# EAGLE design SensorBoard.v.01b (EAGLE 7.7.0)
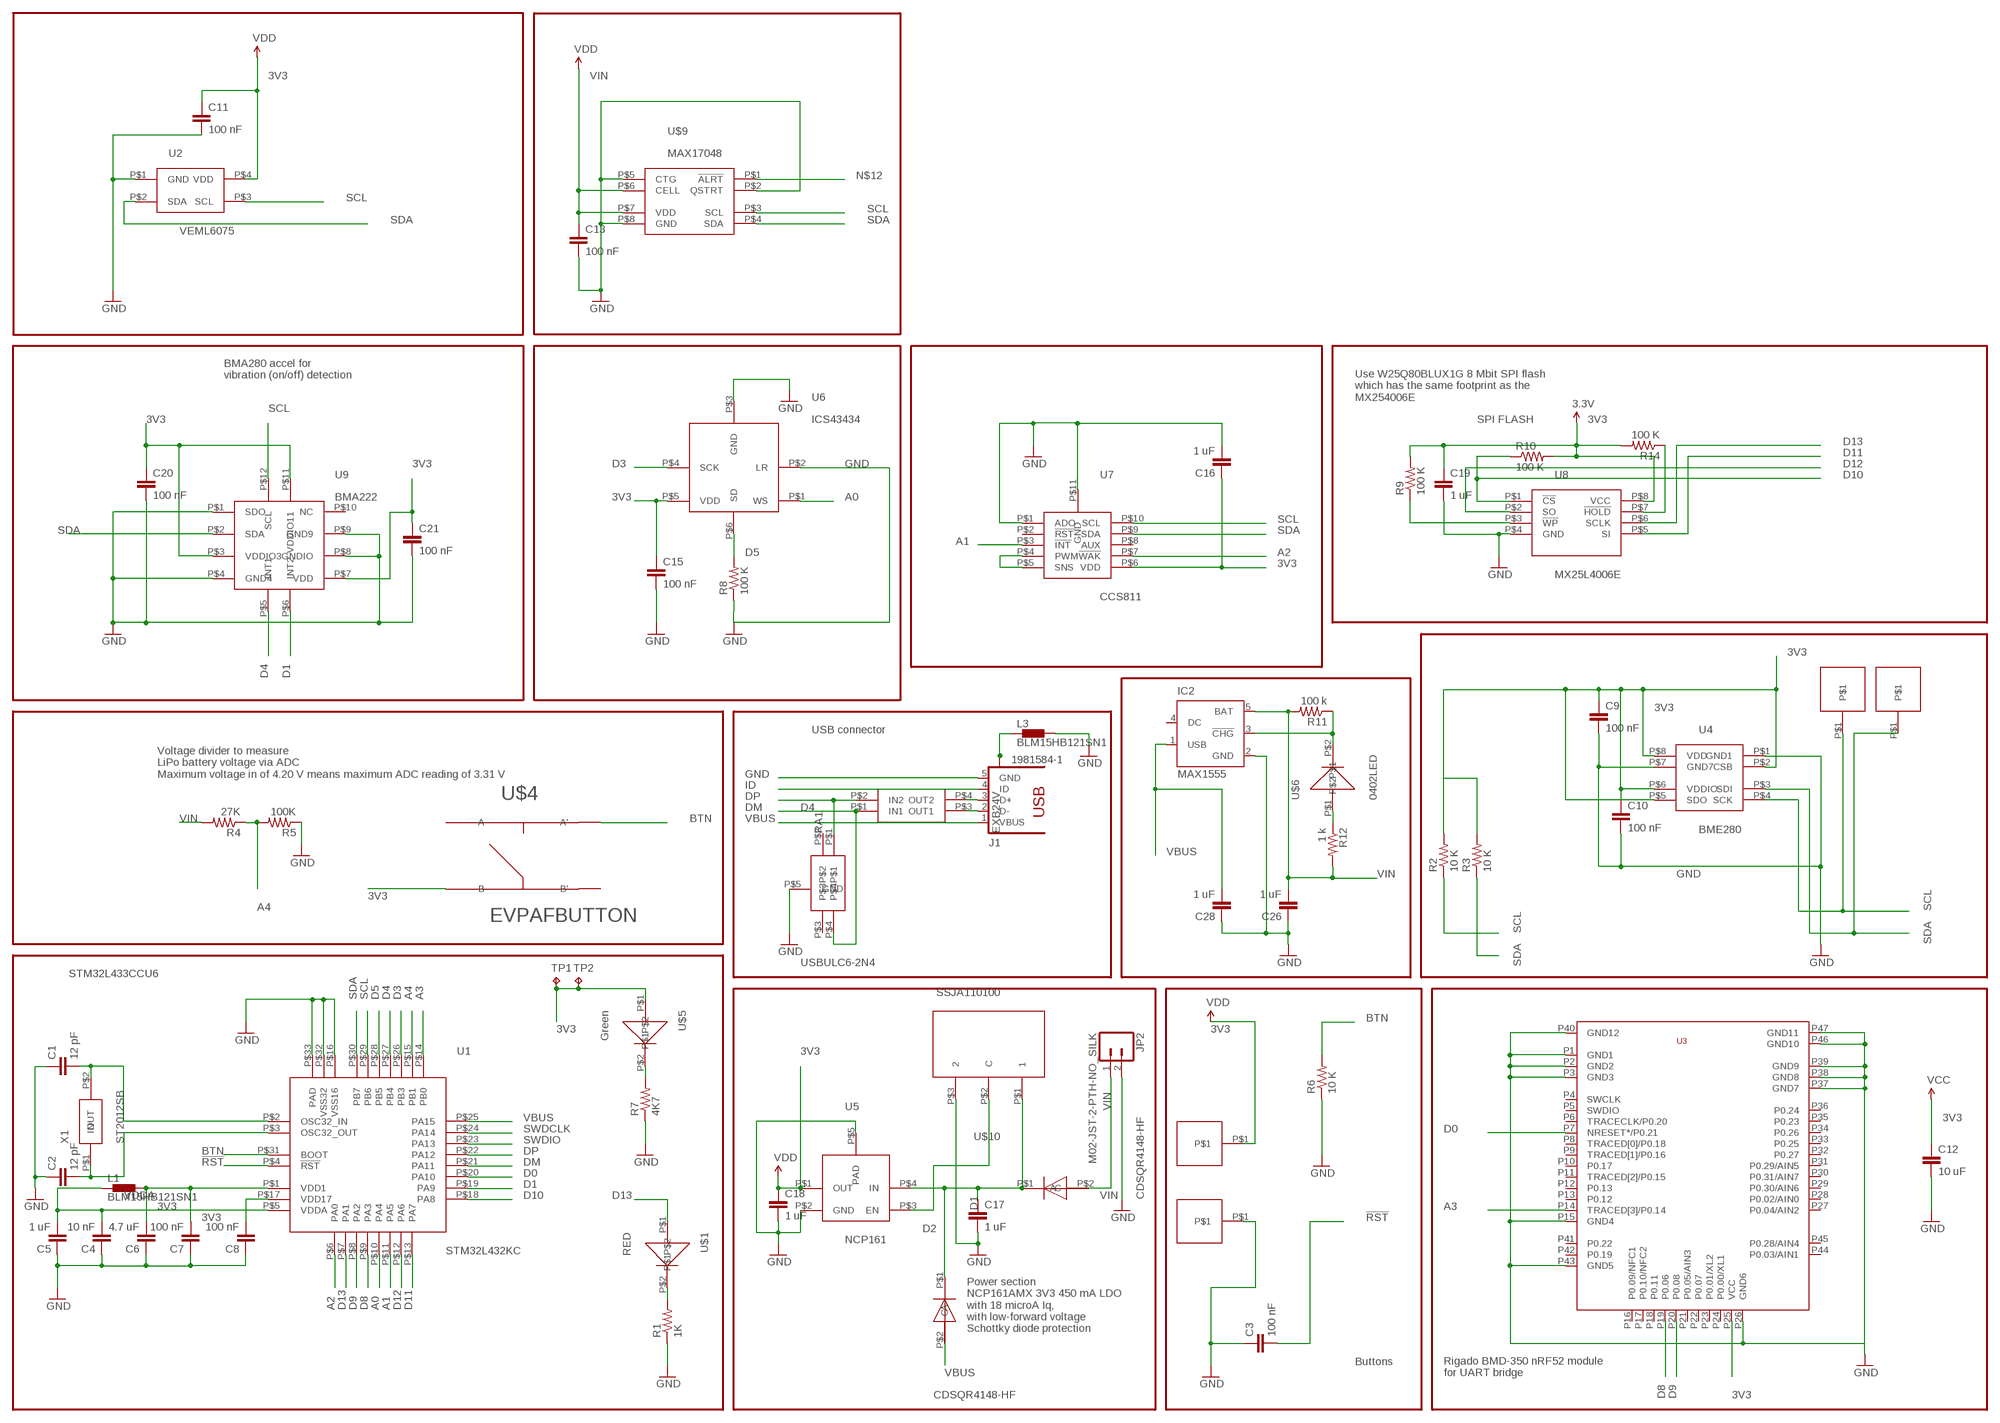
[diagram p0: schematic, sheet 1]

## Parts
C1  12 pF  0402CAP.KW  [0402-CAP]
C2  12 pF  0402CAP.KW  [0402-CAP]
C3  100 nF  0402CAP.KW  [0402-CAP]
C4  10 nF  0402CAP.KW  [0402-CAP]
C5  1 uF  0402CAP.KW  [0402-CAP]
C6  4.7 uF  0402CAP.KW  [0402-CAP]
C7  100 nF  0402CAP.KW  [0402-CAP]
C8  100 nF  0402CAP.KW  [0402-CAP]
C9  100 nF  CAP0402-CAP  [0402-CAP]
C10  100 nF  CAP0402-CAP  [0402-CAP]
C11  100 nF  0402CAP.KW  [0402-CAP]
C12  10 uF  CAP0402-CAP  [0402-CAP]
C13  100 nF  0402CAP.KW  [0402-CAP]
C15  100 nF  0402CAP.KW  [0402-CAP]
C16  1 uF  0402CAP.KW  [0402-CAP]
C17  1 uF  0402CAP.KW  [0402-CAP]
C18  1 uF  0402CAP.KW  [0402-CAP]
C19  1 uF  0402CAP.KW  [0402-CAP]
C20  100 nF  CAP0402-CAP  [0402-CAP]
C21  100 nF  CAP0402-CAP  [0402-CAP]
C26  1 uF  0402CAP.KW  [0402-CAP]
C28  1 uF  0402CAP.KW  [0402-CAP]
D1  CDSQR4148-HF  [CDSQR4148-HF]
D2  CDSQR4148-HF  [CDSQR4148-HF]
D4  USBULC6-2N4  [USBULC6-2N4]
IC2  MAX1555  [SOT23-5L]
J1  1981584-1  [1981584-1]
JP2  M02-JST-2-PTH-NO_SILK  [JST-2-PTH-NS]
L1  BLM15HB121SN1  [0402]
L3  BLM15HB121SN1  [0402]
R1  1K  0402RES.KW  [0402-RES]
R2  10 K  0402RES.KW  [0402-RES]
R3  10 K  0402RES.KW  [0402-RES]
R4  27K  0402RES.KW  [0402-RES]
R5  100K  0402RES.KW  [0402-RES]
R6  10 K  0402RES.KW  [0402-RES]
R7  4K7  0402RES.KW  [0402-RES]
R8  100 K  0402RES.KW  [0402-RES]
R9  100 K  0402RES.KW  [0402-RES]
R10  100 K  0402RES.KW  [0402-RES]
R11  100 k  0402RES.KW  [0402-RES]
R12  1 k  0402RES.KW  [0402-RES]
R14  100 K  0402RES.KW  [0402-RES]
RA1  EXB24V  [EXB24V]
TP1  TPTP06SQ  [TP06SQ]
TP2  TPTP06SQ  [TP06SQ]
U1  STM32L432KC  [STM32L432KC]
U2  VEML6075  [A3OP]
U3  BMD-350  [BMD-350]
U4  BME280  [BME280]
U5  NCP161  [NCP161]
U6  ICS43434  [ICS43434]
U7  CCS811  [CCS811]
U8  MX25L4006E  [USON-8]
U9  BMA222  [BMA222]
U$1  RED  0402LED  [0402LED]
U$2  HN01  [HN01]
U$3  HN01  [HN01]
U$4  EVPAFBUTTON  [EVPAF-BUTTON-SPDT]
U$5  Green  0402LED  [0402LED]
U$6  0402LED  [0402LED]
U$7  HN01  [HN01]
U$8  HN01  [HN01]
U$9  MAX17048  [MAX17048]
U$10  SSJA110100  [SSAJ110100]
X1  ST2012SB  [ST2012SB]

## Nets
3V3: C6.2 C7.2 C8.2 C9.1 C10.1 C11.1 C12.1 C15.1 C16.1 C18.1 C19.1 C20.1 C21.1 L1.2 R2.2 R3.2 R9.2 R10.2 R14.2 TP1.TP TP2.TP U1.P$1(VDD1) U1.P$17(VDD17) U2.P$4(VDD) U3.P25(VCC) U4.P$2(CSB) U4.P$5(SDO) U4.P$6(VDDIO) U4.P$8(VDD) U5.P$1(OUT) U6.P$5(VDD) U7.P$6(VDD) U8.P$8(VCC) U9.P$3(VDDIO3) U9.P$7(VDD) U9.P$11(VDDIO11) U$2.P$1 U$4.P$3(B) U$5.P$1 ; supply symbol labelled VDD, VCC, 3.3V
!RST: C3.2 U1.P$4(!RST)
A0: U1.P$10(PA4) U6.P$1(WS)
A1: U1.P$11(PA5) U7.P$3(!INT)
A2: U1.P$6(PA0) U7.P$7(!WAK)
A3: U1.P$14(PB0) U3.P14(TRACED[3]/P0.14)
A4: R4.1 R5.2 U1.P$15(PB1)
BTN: R6.2 U1.P$31(BOOT) U$4.P$2(A')
D0: U1.P$20(PA10) U3.P7(NRESET*/P0.21)
D1: U1.P$19(PA9) U9.P$6(INT2)
D3: U1.P$26(PB3) U6.P$4(SCK)
D4: U1.P$27(PB4) U9.P$5(INT1)
D5: R8.2 U1.P$28(PB5) U6.P$6(SD)
D8: U1.P$9(PA3) U3.P19(P0.06)
D9: U1.P$8(PA2) U3.P20(P0.08)
D10: R10.1 U1.P$18(PA8) U8.P$1(!CS)
D11: U1.P$13(PA7) U8.P$5(SI)
D12: U1.P$12(PA6) U8.P$2(SO)
D13: U1.P$7(PA1) U8.P$6(SCLK) U$1.P$1
DM: D4.P$4 RA1.P$1(IN1) U1.P$21(PA11)
DP: D4.P$1 RA1.P$2(IN2) U1.P$22(PA12)
GND: C1.1 C2.1 C3.1 C4.1 C5.1 C6.1 C7.1 C8.1 C9.2 C10.2 C11.2 C12.2 C13.2 C15.2 C16.2 C17.2 C18.2 C19.2 C20.2 C21.2 C26.1 C28.1 D4.P$5(GND) IC2.2(GND) J1.5(GND) JP2.2 L3.2 R1.1 R5.1 R6.1 R7.1 R8.1 U1.P$16(VSS16) U1.P$32(VSS32) U1.P$33(PAD) U2.P$1(GND) U3.P1(GND1) U3.P2(GND2) U3.P3(GND3) U3.P15(GND4) U3.P26(GND6) U3.P37(GND7) U3.P38(GND8) U3.P39(GND9) U3.P40(GND12) U3.P43(GND5) U3.P46(GND10) U3.P47(GND11) U4.P$1(GND1) U4.P$7(GND7) U5.P$2(GND) U5.P$5(PAD) U6.P$2(LR) U6.P$3(GND) U7.P$1(ADO) U7.P$11(GND) U8.P$4(GND) U9.P$1(SDO) U9.P$4(GND4) U9.P$8(GNDIO) U9.P$9(GND9) U$3.P$1 U$9.P$2(QSTRT) U$9.P$5(CTG) U$9.P$8(GND) U$10.P$3
ID: J1.4(ID)
N$1: R1.2 U$1.P$2
N$2: U5.P$3(EN) U$10.P$2(C)
N$3: C1.2 U1.P$2(OSC32_IN) X1.P$2(OUT)
N$4: C2.2 U1.P$3(OSC32_OUT) X1.P$1(IN)
N$7: R7.2 U$5.P$2
N$10: U7.P$4(PWM) U7.P$5(SNS)
N$12: U$9.P$1(!ALRT)
N$20: R9.1 U8.P$3(!WP)
N$21: R14.1 U8.P$7(!HOLD)
N$31: J1.3(D+) RA1.P$4(OUT2)
N$33: J1.2(D-) RA1.P$3(OUT1)
N$43: R12.1 U$6.P$1
N$48: IC2.3(!CHG) R11.1 U$6.P$2
N$60: C17.1 D1.P$1(C) D2.P$1(C) U5.P$4(IN) U$10.P$1
SCL: R2.1 U1.P$29(PB6) U2.P$3(SCL) U4.P$4(SCK) U7.P$10(SCL) U9.P$12(SCL) U$7.P$1 U$9.P$3(SCL)
SDA: R3.1 U1.P$30(PB7) U2.P$2(SDA) U4.P$3(SDI) U7.P$9(SDA) U9.P$2(SDA) U$8.P$1 U$9.P$4(SDA)
SWDCLK: U1.P$24(PA14)
SWDIO: U1.P$23(PA13)
USB_SHIELD: J1.S1 J1.S2 J1.S3 J1.S4 L3.1
VBUS: C28.2 D2.P$2(A) IC2.1(USB) J1.1(VBUS) U1.P$25(PA15)
VDDA: C4.2 C5.2 L1.1 U1.P$5(VDDA)
VIN: C13.1 C26.2 D1.P$2(A) IC2.5(BAT) JP2.1 R4.2 R11.2 R12.2 U$9.P$6(CELL) U$9.P$7(VDD) ; supply symbol labelled VDD
Unconnected: D4.P$2 D4.P$3 IC2.4(DC) U3.P4(SWCLK) U3.P5(SWDIO) U3.P6(TRACECLK/P0.20) U3.P8(TRACED[0]/P0.18) U3.P9(TRACED[1]/P0.16) U3.P10(P0.17) U3.P11(TRACED[2]/P0.15) U3.P12(P0.13) U3.P13(P0.12) U3.P16(P0.09/NFC1) U3.P17(P0.10/NFC2) U3.P18(P0.11) U3.P21(P0.05/AIN3) U3.P22(P0.07) U3.P23(P0.01/XL2) U3.P24(P0.00/XL1) U3.P27(P0.04/AIN2) U3.P28(P0.02/AIN0) U3.P29(P0.30/AIN6) U3.P30(P0.31/AIN7) U3.P31(P0.29/AIN5) U3.P32(P0.27) U3.P33(P0.25) U3.P34(P0.26) U3.P35(P0.23) U3.P36(P0.24) U3.P41(P0.22) U3.P42(P0.19) U3.P44(P0.03/AIN1) U3.P45(P0.28/AIN4) U7.P$2(!RST) U7.P$8(AUX) U9.P$10(NC) U$4.P$1(A) U$4.P$4(B')

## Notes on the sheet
- BMA280 accel for
  vibration (on/off) detection
- Use W25Q80BLUX1G 8 Mbit SPI flash 
  which has the same footprint as the 
  MX254006E
- SPI FLASH
- USB connector
- Voltage divider to measure 
  LiPo battery voltage via ADC
  Maximum voltage in of 4.20 V means maximum ADC reading of 3.31 V
- STM32L433CCU6
- Power section
  NCP161AMX 3V3 450 mA LDO
  with 18 microA Iq, 
  with low-forward voltage 
  Schottky diode protection
- Buttons
- Rigado BMD-350 nRF52 module
  for UART bridge

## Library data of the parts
C1-C8 C11 C13 C15-C19 C26 C28 = SparkFun-Capacitors:0402CAP.KW
C9 C10 C12 C20 C21 = SparkFun-Capacitors:CAP: Capacitor
D1 D2 = Kris:CDSQR4148-HF: ComChip's CDSQR4148-HF high speed 150 mA Io diode
D4 = Kris:USBULC6-2N4: ST TVS diode ESD Protection USBULC6-2N4
IC2 = maxim:MAX1555: Dual-Input USB/AC Adapter 1-Cell Li+ Battery Chargers Source: http://www.maxim-ic.com .. MAX1551-MAX1555.pdf; MF: MAXIM; MPN: MAX1555EZK+T; OC_FARNELL: 1628222; OC_NEWARK: 59J2761
J1 = con-usb:1981584-1: Receptacle, micro-USB, type A/B Tyco Electronics; MF: Hirose; MPN: ZX62-AB-5PA(11)
JP2 = SparkFun-Connectors:M02: Standard 2-pin 0.1" header. Use with
L1 L3 = inductors:BLM15H: EMIFIL (R) Chip Ferrite Bead for GHz Noise
R1-R12 R14 = SparkFun-Resistors:0402RES.KW
RA1 = Kris:EXB24V: Panasonic EXB24 22 Ohm series resistor pair
TP1 TP2 = testpad:TP: Test pad
U1 = STM32L432KC:STM32L432KC: STM32L432KC UFQFPN32 - 32-pin, 5x5 mm, 0.5 mm pitch ultra thin fine pitch quad flat package http://www.st.com/content/ccc/resource/technical/document/datasheet/24/01/9f/59/f0/83/47/fc/DM00257205.pdf/files/DM00257205.pdf/jcr:content/translations/en.DM00257205.pdf
U2 = Kris:VEML6075: A3OP package for VEML6040 and VEML6075 Vishay light sensors
U3 = BMD-350-Eagle:BMD-350
U4 = Kris:BME280: BME280 Bosch pressure, humidity, temperature sensor
U5 = Kris:NCP161: NCP161 3V3 LDO voltage regulator
U6 = Invensense:ICS43434: ICS43434 I2S Digital Microphone
U7 = Kris:CCS811: CCS811 Air Quality Sensor http://ams.com/eng/Products/Environmental-Sensors/Gas-Sensors/CCS811
U8 = Kris:MX25L4006E: uson-8 package for Macronix MX25L4006E 4 Mbit SPI Fash
U9 = Kris:BMA222: Bosch BMA222 3-axis accelerometer
U$1 U$5 U$6 = Kris:0402LED: 0402led
U$2 U$3 U$7 U$8 = PWSONN6:HN01
U$4 = SparkFun-Electromechanical:EVPAFBUTTON: EVPAF Momentary switch by panasonic
U$9 = Kris:MAX17048: MAX17048 LiPo Battery Fuel Gauge
U$10 = Kris:SSJA110100: ALPS SSJA110100 SPDT slide switch with lugs
X1 = Kris:ST2012SB: Kyocera 2.0 x 1.2 mm 32.768 20kHz ppm 4 pf crystal

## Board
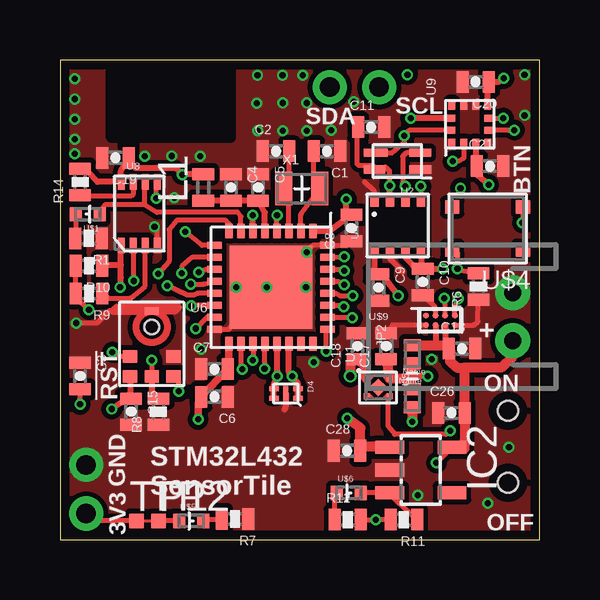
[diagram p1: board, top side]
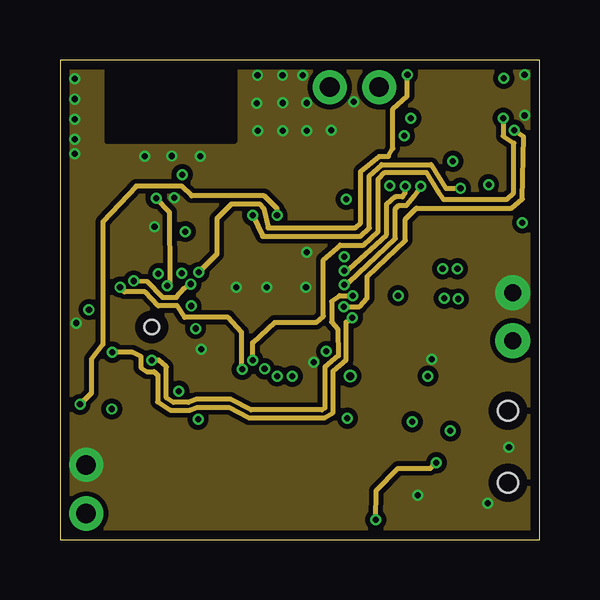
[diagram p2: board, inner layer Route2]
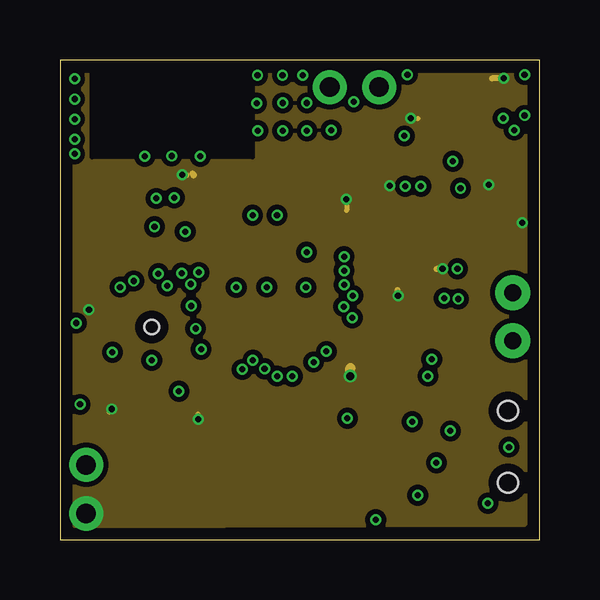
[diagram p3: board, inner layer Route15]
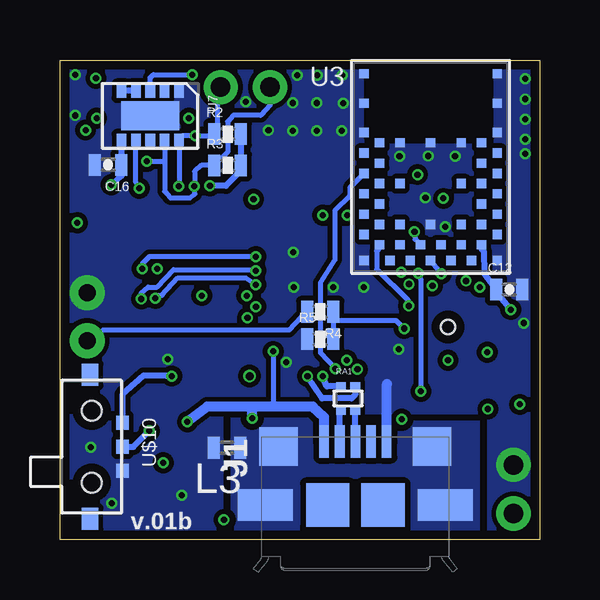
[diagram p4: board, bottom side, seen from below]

Size 19.99 x 19.99 mm. Coordinates in mm from the lower left corner, seen from the top.
Outline: 0,0 19.99,0 19.99,19.99 0,19.99 0,0
Copper layers (1*2*15*16): Top 0.035559375mm / dielectric 0.17018125mm / Route2 0.01778125mm / dielectric 47mil / Route15 0.01778125mm / dielectric 0.17018125mm / Bottom 0.035559375mm
Design rules "OSHPark-4layer *": minimum track width 5mil, minimum drill 10mil, track to track 5mil, track to pad 5mil, pad to pad 5mil, via to via 5mil, smd to smd 5mil, copper to edge 15mil, drill to drill 6mil, minimum pad ring 4mil, minimum via ring 4mil, stop-mask expansion 4mil, vias tented up to drill 20mil, thermal gap 10mil

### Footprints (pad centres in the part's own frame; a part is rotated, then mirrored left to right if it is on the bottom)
0402-CAP = smd 0.5 x 0.9: 1 -0.55,0; 2 0.55,0
CDSQR4148-HF = smd 0.7 x 0.5: P$1 0,0.375; P$2 0,-0.375
USBULC6-2N4 = smd 0.2 x 0.4: P$1 0.2,0.5; P$2 -0.2,0.5; P$3 -0.2,-0.5; P$4 0.2,-0.5 | smd 0.6 x 0.2: P$5 0,0
SOT23-5L = smd 0.55 x 1.2: 1 -0.95,-1.3; 2 0,-1.3; 3 0.95,-1.3; 4 0.95,1.3; 5 -0.95,1.3
1981584-1 = smd 0.4 x 1.35: 1 -1.3,4.1; 2 -0.65,4.1; 3 0,4.1; 4 0.65,4.1; 5 1.3,4.1 | smd 1.8 x 1.8: M1 -1.15,1.45; M2 1.15,1.45 | smd 2.3 x 1.3: S1 -3.75,1.45; S2 3.75,1.45 | smd 1.6 x 1.6: S3 -3.2,3.885; S4 3.2,3.885
JST-2-PTH-NS = drill 0.7 pad 1.448: 1 -1,0; 2 1,0
0402 = smd 0.5 x 0.9: 1 -0.55,0; 2 0.55,0
0402-RES = smd 0.5 x 0.9: 1 -0.55,0; 2 0.55,0
EXB24V = smd 0.4 x 0.36: P$1 -0.3,0.5; P$2 0.3,0.5; P$3 -0.3,-0.5; P$4 0.3,-0.5
TP06SQ = smd 0.6 x 0.6: TP 0,0
STM32L432KC = smd 0.6 x 0.3: P$1 -2.35,1.75; P$2 -2.35,1.25; P$3 -2.35,0.75; P$4 -2.35,0.25; P$5 -2.35,-0.25; P$6 -2.35,-0.75; P$7 -2.35,-1.25; P$8 -2.35,-1.75; P$17 2.35,-1.75; P$18 2.35,-1.25; P$19 2.35,-0.75; P$20 2.35,-0.25; P$21 2.35,0.25; P$22 2.35,0.75; P$23 2.35,1.25; P$24 2.35,1.75 | smd 0.3 x 0.6: P$9 -1.75,-2.35; P$10 -1.25,-2.35; P$11 -0.75,-2.35; P$12 -0.25,-2.35; P$13 0.25,-2.35; P$14 0.75,-2.35; P$15 1.25,-2.35; P$16 1.75,-2.35; P$25 1.75,2.35; P$26 1.25,2.35; P$27 0.75,2.35; P$28 0.25,2.35; P$29 -0.25,2.35; P$30 -0.75,2.35; P$31 -1.25,2.35; P$32 -1.75,2.35 | smd 3.45 x 3.45: P$33 0,0
A3OP = smd 0.9 x 0.35: P$1 -0.95,0.35; P$2 -0.95,-0.35; P$4 0.95,0.35 | smd 1 x 0.35: P$3 0.9,-0.35
BMD-350 = smd 0.39 x 0.39: P1 0.425,8.2; P2 0.425,6.975; P3 0.425,5.75; P4 1.075,5.325; P5 0.425,4.9; P6 1.075,4.475; P7 0.425,4.05; P8 1.075,3.625; P9 0.425,3.2; P10 1.075,2.775; P11 0.425,2.35; P12 1.075,1.925; P13 0.425,1.5; P14 1.075,1.075; P15 0.425,0.425; P16 1.5,0.425; P17 1.925,1.075; P18 2.35,0.425; P19 2.775,1.075; P20 3.2,0.425; P21 3.625,1.075; P22 4.05,0.425; P23 4.475,1.075; P24 4.9,0.425; P25 5.325,1.075; P26 5.975,0.425; P27 5.975,1.5; P28 5.325,1.925; P29 5.975,2.35; P30 5.325,2.775; P31 5.975,3.2; P32 5.325,3.625; P33 5.975,4.05; P34 5.325,4.475; P35 5.975,4.9; P36 5.325,5.325; P37 5.975,5.75; P38 5.975,6.975; P39 5.975,8.2; P40 1.925,5.325; P41 1.925,3.625; P42 1.925,1.925; P43 3.2,1.925; P44 4.475,1.925; P45 4.475,3.625; P46 4.475,5.325; P47 3.2,5.325
BME280 = smd 0.5 x 0.35: P$1 1.025,0.975; P$2 1.025,0.325; P$3 1.025,-0.325; P$4 1.025,-0.975; P$5 -1.025,-0.975; P$6 -1.025,-0.325; P$7 -1.025,0.325; P$8 -1.025,0.975
NCP161 = smd 0.24 x 0.24: P$1 -0.37,-0.48; P$2 0.37,-0.48; P$3 0.37,0.48; P$4 -0.37,0.48 | smd 0.52 x 0.52 rotated 45: P$5 0,0
ICS43434 = smd 0.6 x 0.522: P$1 0.9,-1.364; P$2 0.9,-0.532; P$4 -0.9,-0.532; P$5 -0.9,-1.364; P$6 0,-1.364 | smd 0.6 x 0.3: P$3 0,1.368 | hole 0.6: 0,0.7
CCS811 = smd 0.6 x 0.4: P$1 -1.05,1.2; P$2 -1.05,0.6; P$3 -1.05,0; P$4 -1.05,-0.6; P$5 -1.05,-1.2; P$6 1.05,-1.2; P$7 1.05,-0.6; P$8 1.05,0; P$9 1.05,0.6; P$10 1.05,1.2 | smd 1.2 x 2.4: P$11 0,0
USON-8 = smd 0.3 x 0.65: P$1 -0.75,-1.325; P$2 -0.25,-1.325; P$3 0.25,-1.325; P$4 0.75,-1.325; P$5 0.75,1.325; P$6 0.25,1.325; P$7 -0.25,1.325; P$8 -0.75,1.325
BMA222 = smd 0.41 x 0.28: P$1 -0.815,0.75; P$2 -0.815,0.25; P$3 -0.815,-0.25; P$4 -0.815,-0.75; P$7 0.815,-0.75; P$8 0.815,-0.25; P$9 0.815,0.25; P$10 0.815,0.75 | smd 0.28 x 0.41: P$5 -0.25,-0.815; P$6 0.25,-0.815; P$11 0.25,0.815; P$12 -0.25,0.815
0402LED = smd 0.5 x 0.6: P$1 -0.5,0; P$2 0.5,0
HN01 = drill 0.813 pad 1.422: P$1 0,0
EVPAF-BUTTON-SPDT = smd 0.6 x 0.55: P$1 -1.475,0.9; P$2 1.475,0.9; P$3 -1.475,-0.9; P$4 1.475,-0.9
MAX17048 = smd 0.25 x 0.25: P$1 -0.6,0.2; P$2 -0.2,0.2; P$3 0.2,0.2; P$4 0.6,0.2; P$5 -0.6,-0.2; P$6 -0.2,-0.2; P$7 0.2,-0.2; P$8 0.6,-0.2
SSAJ110100 = smd 0.6 x 0.51: P$1 -1,1.28; P$2 0,1.285; P$3 1,1.285 | smd 0.9 x 0.7: P$4 3,-0.07; P$5 -3,-0.07 | hole 0.83: -1.5,0; 1.5,0
ST2012SB = smd 0.7 x 1.4: P$1 -0.75,0; P$2 0.75,0

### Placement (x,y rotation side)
C1  11.13,16.19 180 top
C2  9,16.19 0 top
C3  0.84,6.82 270 top
C4  7.12,14.68 270 top
C5  8.26,14.68 270 top
C6  6.44,5.96 180 top
C7  6.44,7.11 0 top
C8  12.14,12.99 90 top
C9  13.27,10.5 270 top
C10  15.11,10.74 270 top
C11  12.97,17.2 0 top
C12  1.27,10.43 0 bottom
C13  16.75,7.96 0 top
C15  2.96,5.33 270 top
C16  17.98,15.62 180 bottom
C17  13.59,8.06 90 top
C18  12.4,8.06 90 top
C19  2.31,15.91 180 top
C20  17.32,19.08 180 top
C21  17.92,15.57 0 top
C26  16.31,5.28 0 top
C28  11.96,3.71 0 top
D1  14.68,7.73 180 top
D2  14.68,5.91 0 top
D4  9.41,6.1 270 top
IC2  15.04,2.91 270 top
J1  7.68,0 0 bottom
JP2  18.86,9.3 90 top
L1  5.97,14.68 90 top
L3  13.03,3.84 180 bottom
R1  1.19,12.56 180 top
R2  13,16.9 0 bottom
R3  13,15.6 0 bottom
R4  9.14,9.5 180 bottom
R5  9.14,8.36 0 bottom
R6  17.44,10.55 90 top
R7  7.29,0.86 180 top
R8  4.1,5.33 90 top
R9  1.21,10.26 180 top
R10  1.21,11.42 180 top
R11  14.33,0.84 180 top
R12  11.99,0.84 0 top
R14  0.84,14.91 90 top
RA1  7.99,5.89 0 bottom
TP1  3.19,0.79 0 top
TP2  4.1,0.79 0 top
U1  8.79,10.52 270 top
U2  14.06,15.77 180 top
U3  7.75,11.21 0 bottom
U4  14.07,13.09 90 top
U5  13.26,6.35 270 top
U6  3.82,8.17 0 top
U7  16.23,17.67 270 bottom
U8  3.3,13.59 0 top
U9  17.07,17.31 90 top
U$1  1.16,13.56 180 top
U$2  1.09,1.09 90 top
U$3  1.09,3.12 0 top
U$4  17.82,12.97 180 top
U$5  5.47,0.79 0 top
U$6  12.04,1.96 0 top
U$7  13.3,18.86 0 top
U$8  11.24,18.86 0 top
U$9  15.85,9.14 0 top
U$10  18.67,3.87 270 bottom
X1  10.07,14.63 0 top

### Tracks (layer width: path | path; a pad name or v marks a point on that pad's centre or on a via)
3V3  (via drill 0.25, 0.33)
  Top 0.127: TP1.TP TP2.TP
  Top 0.203: C8.2 11.92,13.65 | C6.2 5.76,5.68 | 13.75,14.61 v13.74,14.74 13.73,14.86 13.73,15.38 13.57,15.53 U2.P$4 13.05,15.6 R3.2 12.38,15.66 12.38,17.04 C11.1 | 15.05,11.33 15.08,11.33 C10.1 | v1.21,9.59 0.66,10.1 R9.2 R10.2 | C19.1 2.86,15.77 | 1.18,15.3 0.93,15.33 R14.2 | TP1.TP 1.4,0.79 U$2.P$1 | U$5.P$1 TP2.TP | U$4.P$3 19.29,13.96
  Top 0.254: 11.92,13.65 v11.93,14.19 | U1.P$1 11.25,12.87 C8.2 | C7.2 6.95,7.09 | L1.2 5.05,15.23 v5.09,15.21 4.83,15.49 3.15,15.49 2.86,15.77 | U4.P$8 13.1,11.21 C9.1 13.41,11.05 v14.08,10.17 | U4.P$6 14.41,11.75 14.9,11.23 C10.1 15.82,11.29 v15.94,11.29 | U4.P$2 13.75,14.61 | U4.P$5 15.05,11.33 | 13.72,14.77 v13.74,14.74 | v2.16,5.45 2.92,5.93 C15.1 2.92,6.11 U6.P$5 | C19.1 2.54,15.36 U8.P$8 1.56,14.91 1.18,15.3 | v18.49,19.23 18.27,19.07 C20.1 17.82,18.88 U9.P$7 | U9.P$3 17.32,16.02 C21.1 17.37,15.23 v17.86,14.8 | U9.P$11 v14.62,17.56 | 19.29,13.96 19.29,13.23 v19.27,13.21
  Top 0.305: 5.76,5.68 v5.75,5.02 | C6.2 6.95,7.09 7.04,7.17 7.04,7.67 U1.P$17
  Top 0.406: U5.P$1 12.74,6.81 12.74,6.92 12.74,7.22 C18.1 12.2,7.54 12.1,7.39 12.1,6.86 v12.09,6.82
  Route15 0.203: v11.93,14.19 11.94,13.73 | v5.75,5.02 5.75,5.23 | v13.74,14.74 13.66,14.77 13.68,14.72 | v14.62,17.56 14.91,17.55
  Route15 0.254: v5.09,15.21 4.99,15.2 5.27,15.2 | 5.56,15.18 5.59,15.2 5.58,15.2 5.52,15.25 | v1.21,9.59 1.21,9.68 | v14.08,10.17 14.07,10.41 | v15.94,11.29 15.7,11.29 | v2.16,5.45 2.06,5.33 | v18.49,19.23 18.01,19.23 | v19.27,13.21 19.27,13.17 19.28,13.13
  Route15 0.406: v12.09,6.82 12.1,7.16
  Bottom 0.203: 17.43,16.06 17.44,15.46
  Bottom 0.254: v1.21,9.59 1.88,10.39 C12.1 2.31,11.09 2.32,12.01 2.42,12.12 U3.P25 | R2.2 R3.2 12.46,15.37 13.08,14.74 v13.74,14.74 | U7.P$6 17.43,16.06 C16.1 | 17.44,15.46 17.44,15.16 v17.86,14.8
  pour Route15 (isolate 0.203, no thermals): 0.64,19.35 19.35,19.35 19.35,0.64 0.64,0.57
!RST  (via drill 0.25)
  Top 0.203: U1.P$4 v9.04,13.52 v9.04,13.53 | C3.2 0.81,5.85 v0.83,5.64
  Route2 0.203: v9.04,13.53 9.04,13.79 8.51,14.33 5.49,14.33 5.07,14.73 3.17,14.73 1.79,13.26 1.79,8.14 1.31,7.53 1.31,6.11 v0.83,5.64
A0  (via drill 0.25)
  Top 0.203: U1.P$10 5.5,11.77 5.08,11.39 v5.07,11.1 | v4.95,6.18 4.95,6.57 U6.P$1
  Bottom 0.203: v5.07,11.1 4.95,10.83 v4.95,6.18
A1  (via drill 0.25)
  Top 0.203: U1.P$11 6.12,11.27 v5.78,11.14
  Route2 0.203: v14.48,19.38 14.46,19.23 14.46,18.49 13.87,17.96 13.87,16.31 13.68,15.98 13.3,15.98 12.52,15.35 12.52,13.21 12.29,12.99 8.67,12.99 8.48,13.79 8.31,13.99 7.15,13.99 6.54,13.37 6.54,11.9 v5.78,11.14
  Bottom 0.203: U7.P$3 16.23,19.25 16.1,19.38 v14.48,19.38
A2  (via drill 0.25)
  Top 0.254: U1.P$6 8.04,13.46 v8.03,13.53
  Route2 0.203: v8.03,13.53 8.45,12.64 12.51,12.64 12.89,12.99 12.89,15.18 13.4,15.63 15.47,15.63 16.08,14.64 v16.69,14.64
  Bottom 0.203: U7.P$7 16.83,14.89 v16.69,14.64
A3  (via drill 0.25)
  Top 0.203: U1.P$14 5.59,9.77 v5.46,9.74
  Bottom 0.203: U3.P14 6.67,12.18 6.79,12.03 6.79,11.27 5.47,9.97 v5.46,9.74
A4  (via drill 0.25)
  Top 0.203: U1.P$15 6.11,9.27 v5.65,8.8
  Bottom 0.203: R5.2 R4.1 8.55,9.41 8.37,9.13 5.99,9.13 v5.65,8.8
BTN  (via drill 0.25)
  Top 0.203: U1.P$31 11.66,11.76 v11.84,11.8 | U$4.P$2 16.34,12.16 16.56,11.94 v16.56,11.29 16.6,11.26 R6.2
  Bottom 0.203: v11.84,11.8 16.27,11.8 16.56,11.51 v16.56,11.29
D0  (via drill 0.25)
  Top 0.203: v8.52,7.12 8.53,7.33 U1.P$20
  Bottom 0.203: v8.52,7.12 9.14,7.79 9.14,10.72 8.53,11.66 8.53,13.73 7.9,14.36 7.9,14.69 U3.P7
D1  (via drill 0.25)
  Top 0.203: U1.P$19 8.05,7.67 v8.04,7.48 | U9.P$6 v18.47,17.56
  Route2 0.203: v8.04,7.48 8.03,8.22 8.94,9.05 10.67,9.05 10.97,9.32 10.97,11.66 11.67,12.28 12.64,12.28 13.26,12.85 13.26,15.01 13.54,15.3 15.27,15.3 15.75,14.53 15.98,14.19 18.61,14.19 18.9,14.45 18.91,16.52 18.47,16.82 v18.47,17.56
D3  (via drill 0.25)
  Top 0.203: v12.18,9.25 11.16,9.25 U1.P$26 | U6.P$4 2.56,7.63 v2.18,7.81
  Route2 0.203: v12.18,9.25 11.93,9.07 11.93,7.49 11.38,7.04 11.38,5.3 11.02,5.08 7.87,5.08 7.02,5.51 5.71,5.51 5.41,5.4 4.6,5.4 4.06,5.74 4.08,6.86 3.92,7.01 3.61,7.01 3.37,7.18 3.37,7.64 3.04,7.81 v2.18,7.81
D4  (via drill 0.25)
  Top 0.203: U1.P$27 11.61,9.77 v11.82,9.72 | v18.92,17.07 18.68,17.06 U9.P$5
  Route2 0.203: v11.82,9.72 12.48,9.72 12.8,10.06 12.8,10.97 14.39,12.47 14.39,13.36 14.85,13.82 18.81,13.82 19.27,14.2 19.32,16.79 v18.92,17.07
D5  (via drill 0.25)
  Top 0.203: U1.P$28 11.5,10.27 11.65,10.17 v12.21,10.17 | v3.82,7.48 U6.P$6
  Top 0.254: U6.P$6 3.82,6.09 R8.2
  Route2 0.203: v3.82,7.48 4.12,7.48 4.43,7.2 4.43,5.91 4.73,5.73 5.35,5.73 5.69,5.86 7.11,5.86 7.96,5.41 10.92,5.41 11.04,5.5 11.04,7.19 11.6,7.66 11.58,8.76 11.32,9.07 11.32,9.93 11.65,10.17 v12.21,10.17
D8  (via drill 0.25)
  Top 0.203: U1.P$9 5.92,12.27 v5.22,12.84
  Bottom 0.203: v5.22,12.84 5.19,12.51 U3.P19
D9  (via drill 0.25)
  Top 0.203: U1.P$8 7.04,13.17 6.91,13.31 4.86,13.31 4.55,12.93 4.55,11.6 v4.1,11.09
  Bottom 0.203: U3.P20 4.55,11.6 v4.1,11.09
D10  (via drill 0.25)
  Top 0.203: U1.P$18 7.54,7.19 v7.59,7.1 | 2.54,12.04 U8.P$1 | R10.1 1.99,11.46
  Top 0.254: v2.5,10.53 2.54,10.92 2.54,11.46 | 2.54,11.46 2.54,12.04 | 1.99,11.46 2.54,11.46
  Route2 0.203: v2.5,10.53 2.68,10.32 3.54,10.32 4.1,9.74 4.88,9.75 5.19,9.27 7.01,9.27 7.57,8.65 7.57,7.09 v7.59,7.1
D11  (via drill 0.25)
  Top 0.203: v4.01,14.22 4.03,14.89 U8.P$5 | U1.P$13 5.76,10.27 5.58,10.2 5.31,10.2 v4.47,10.58
  Route2 0.203: v4.47,10.58 4.58,10.73 4.58,10.85 4.57,13.64 v4.01,14.22
D12  (via drill 0.25)
  Top 0.203: U8.P$2 3.05,10.84 v3.07,10.78 | v5.45,10.65 5.97,10.65 U1.P$12
  Route2 0.203: v3.07,10.78 3.62,10.77 4.27,10.1 4.85,10.1 5.21,10.49 v5.45,10.65
D13
  Top 0.203: U1.P$7 7.54,13.47 7.42,13.64 4.04,13.64 3.53,13.96 3.51,13.97 | U$1.P$1 1.75,13.66 1.75,13.76 1.89,13.97 3.51,13.97 | U8.P$6 3.5,14.85 3.5,14 3.51,13.97
DM  (via drill 0.25)
  Top 0.254: D4.P$4 8.91,6.39 v9.04,6.82 | v9.04,6.82 9.05,6.89 9.05,7.03 | 9.05,7.03 9.05,8.16 U1.P$21 | v9.04,6.82 9.06,6.91 9.05,7.03
  Bottom 0.254: RA1.P$1 8.87,6.39 v9.04,6.82
DP  (via drill 0.25)
  Top 0.254: U1.P$22 9.54,6.99 9.91,6.5 D4.P$1 9.91,6.51 v9.68,6.81
  Bottom 0.254: RA1.P$2 7.69,6.04 7.84,5.89 9.06,5.89 v9.68,6.81
GND  (via drill 0.25)
  Top 0.203: U1.P$16 7.04,8.77 v8.61,10.53 10.54,12.27 U1.P$32 11.95,12.27 C8.1 | U4.P$1 13.1,14.51 12.69,14.92 | U4.P$7 13.75,11.7 14.3,11.15 | 2.22,9.53 2.04,9.53 1.54,9.03 v0.67,9.03 | U8.P$4 4.05,12.93 v3.94,13.04 | 15.11,10.17 C10.2 15.65,9.66 U$9.P$2 | U$9.P$5 13.86,8.94 C17.2 | U$9.P$8 17.24,8.94 17.41,9.09 R6.1
  Top 0.254: D4.P$5 9.41,5.59 9.36,5.42
  Top 0.305: U6.P$3 2.22,9.52 | U6.P$3 4.77,9.53 4.93,9.69 2.38,9.69 2.22,9.53
  Bottom 0.406: J1.5 6.37,6.49
  other vias: 3.53,15.98 7.34,10.52 4.65,15.99 5.84,15.98 8.24,17.04 8.19,18.19 8.23,19.35 9.27,19.35 9.28,18.2 9.28,17.04 0.61,19.2 0.61,18.36 0.61,17.53 10.11,19.35 10.29,18.2 10.29,17.04 11.3,17.07 10.27,11.98 10.25,10.52 14.91,1.85 17.83,1.52 4.76,14.25 19.35,17.68 15.49,7.52 19.35,19.38 12.24,18.25 10.57,7.4 5.88,7.94 0.61,16.69 0.61,16.08 18.71,3.86
  pour Top (isolate 0.203, no thermals): 0,19.99 19.99,19.99 19.99,0 0,0
  pour Route2 (isolate 0.203, no thermals): 0,19.99 19.99,19.99 19.99,0 0,0
  pour Bottom (isolate 0.203, no thermals): 2.1,0 0,0 0,19.99 19.99,19.99 19.99,0 13.27,0 13.27,5.33 2.1,5.33
N$1
  Top 0.203: U$1.P$2 0.66,12.57 R1.2
N$2  (via drill 0.25)
  Top 0.203: v16.27,4.53 16.08,4.39 13.95,4.39 13.66,4.75 13.66,5.98 U5.P$3
  Bottom 0.203: 16.3,4.41 v16.27,4.53
  Bottom 0.254: U$10.P$2 16.93,3.87 v16.27,4.53
N$3
  Top 0.203: U1.P$2 10.04,13.56 X1.P$2 10.58,15.16 C1.2
N$4
  Top 0.203: U1.P$3 9.54,14.17 X1.P$1 9.55,15.26 C2.2
N$5
  cutout Route2: 1.97,19.95 7.28,19.96 7.28,16.59 1.97,16.59
N$6
  cutout Route15: 1.88,19.96 8.01,19.96 8.01,15.95 1.33,15.95 1.33,19.94
N$7
  Top 0.203: U$5.P$2 6.19,0.86 R7.2
N$9
  cutout Top (no thermals): 12.83,14.33 15.35,14.33 15.35,11.82 12.83,11.82 12.83,14.31
N$10
  Bottom 0.254: U7.P$4 U7.P$5
N$20
  Top 0.203: R9.1 1.76,10.16 2.02,10.07 2.95,10.07 3.54,10.57 U8.P$3
N$21
  Top 0.203: U8.P$7 3.05,14.41 2.96,14.31 1.13,14.31 R14.1
N$31
  Bottom 0.254: J1.3 7.68,5.27 RA1.P$4
N$33
  Bottom 0.254: J1.2 8.33,5.23 RA1.P$3
N$43
  Top 0.203: R12.1 11.44,1.85 U$6.P$1
N$48
  Top 0.203: U$6.P$2 IC2.3 13.74,1.9 R11.1
N$60  (via drill 0.25)
  Top 0.254: v15.33,6.82 14.91,6.82 14.6,6.81
  Top 0.406: D2.P$1 14.59,6.57 | 14.59,6.57 14.6,6.81 D1.P$1 | 14.59,6.57 14.59,6.72 U5.P$4 13.66,7.31 C17.1
  Bottom 0.254: v15.33,6.82 15.58,6.83 16.52,6.83 17.39,6.06 17.39,4.91 U$10.P$1
SCL  (via drill 0.25)
  Top 0.203: v15.04,14.73 15.04,14.15 U4.P$4 15.06,14.13 | U1.P$29 11.57,10.77 v11.84,10.63 | U9.P$12 14.56,17.06 14.35,16.9 v14.35,16.83 14.35,16.56 13.82,16.12 U2.P$3 | U$9.P$3 16.05,9.98 v16.02,10.06
  Route2 0.203: v11.84,10.63 12.03,10.73 13.97,12.56 13.97,13.79 14.12,13.93 14.44,13.93 14.76,14.32 v15.05,14.72 v15.04,14.73
  Bottom 0.203: v15.04,14.73 v15.03,14.74 U7.P$10 14.92,16.83 v14.35,16.83 13.69,16.83 R2.1 13.55,17.09 13.41,17.23 13.41,18.75 U$7.P$1 | v16.02,10.06 15.96,10.19 15.75,10.19 15.07,10.91 12.24,10.91 v11.84,10.63
  Bottom 0.254: 13.55,16.65 R2.1
SDA  (via drill 0.25)
  Top 0.203: U1.P$30 11.76,11.27 v11.84,11.21 | v14.39,14.73 14.39,14.26 U4.P$3 | 14.39,14.82 v14.39,14.73 | U9.P$2 16.82,15.89 16.6,15.77 16.46,15.76 v16.37,15.77 | U2.P$2 14.43,16.12 14.28,15.98 14.28,14.85 v14.39,14.73 | U$9.P$4 16.45,9.76 v16.6,10.03
  Route2 0.203: v11.84,11.21 12.05,11.29 13.61,12.71 13.61,13.98 13.97,14.29 14.26,14.29 14.38,14.44 v14.39,14.73
  Bottom 0.203: v14.39,14.73 v14.38,14.74 14.38,15.35 14.1,15.6 R3.1 13.01,16.15 13.01,17.42 12.78,17.68 11.63,17.68 11.24,18.12 U$8.P$1 | U7.P$9 15.63,15.77 | 15.63,15.77 15.63,14.51 15.39,14.25 14.57,14.25 14.37,14.4 14.37,14.71 | v16.37,15.77 15.63,15.77 | v16.6,10.03 16.6,10.3 16.33,10.53 15.94,10.53 15.25,11.25 11.87,11.25 v11.84,11.21
  Bottom 0.254: 14.37,14.71 v14.39,14.73
USB_SHIELD
  pour Bottom (isolate 0.254, rank 3, no thermals): 2.6,0 2.6,5.21 12.76,5.21 12.76,0
VBUS  (via drill 0.25)
  Top 0.203: v11.1,7.85 11.1,8.73 U1.P$25
  Top 0.406: 14.54,5.51 D2.P$2 14.68,5.28 v14.68,4.92 | v11.98,5.07 12.51,4.66 C28.2 12.68,3.87 13.72,3.87 IC2.1
  Bottom 0.203: v11.1,7.85 11.1,5.86 11.09,5.55
  Bottom 0.406: J1.1 8.98,5.11 9.45,5.55 11.09,5.55 12.04,5.55 | 12.04,5.55 13.86,5.55 v14.68,4.92 | v11.98,5.07 11.98,5.49 12.04,5.55
VDDA
  Top 0.254: U1.P$5 8.54,13.63 C5.2 C4.2 L1.1
VIN  (via drill 0.25)
  Top 0.203: R11.2 v13.16,0.84 R12.2 | v15.68,3.21 IC2.5 | 16.25,7.9 C13.1
  Top 0.254: U$9.P$7 16.05,8.12 C13.1 | U$9.P$6 15.65,8.13 15.68,8.1
  Top 0.406: IC2.5 16.4,3.8 16.85,3.8 16.86,4.1 C26.2 16.86,7.17 | JP2.1 18.86,7.63 18.38,7.18 16.86,7.18 16.86,7.17 | D1.P$2 15.68,8.1 16,8.1 C13.1 | 16.25,7.9 16.25,7.42 16.54,7.18 16.85,7.18 16.86,7.17
  Route2 0.203: v13.16,0.84 13.17,2.03 14.08,2.97 15.43,2.97 v15.68,3.21
  Bottom 0.203: R4.2 9.93,9.28 10.45,8.74 18.21,8.74 JP2.1

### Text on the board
tPlace: SCL | SDA | BTN | !RST | + | ON | GND | STM32L432 / SensorTile | OFF | 3V3
bPlace: v.01b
